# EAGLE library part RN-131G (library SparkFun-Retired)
Roving Netowrks WiFLy GSX Module
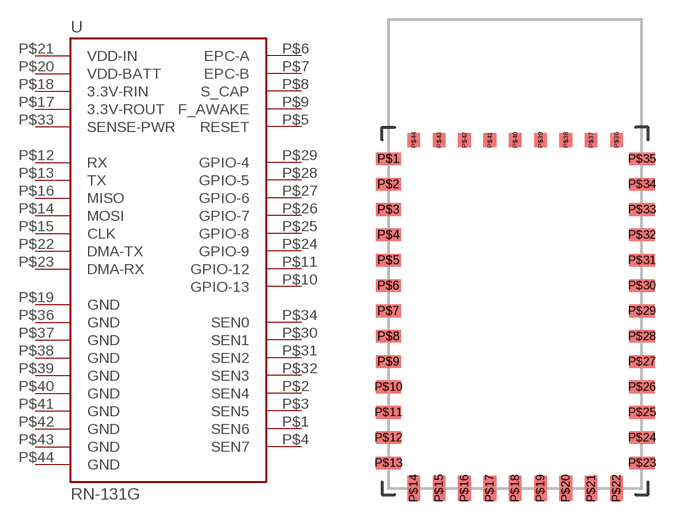
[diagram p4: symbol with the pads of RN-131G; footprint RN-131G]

Designator prefix -

## RN-131G (PROD_ID: IC-12671; SF_ID: WRL-10004)  [RN-131G]
P$1  SEN6
P$2  SEN4
P$3  SEN5
P$4  SEN7
P$5  RESET
P$6  EPC-A
P$7  EPC-B
P$8  S_CAP
P$9  F_AWAKE
P$10  GPIO-13
P$11  GPIO-12
P$12  RX
P$13  TX
P$14  MOSI
P$15  CLK
P$16  MISO
P$17  3.3V-ROUT
P$18  3.3V-RIN
P$19  GND
P$20  VDD-BATT
P$21  VDD-IN
P$22  DMA-TX
P$23  DMA-RX
P$24  GPIO-9
P$25  GPIO-8
P$26  GPIO-7
P$27  GPIO-6
P$28  GPIO-5
P$29  GPIO-4
P$30  SEN1
P$31  SEN2
P$32  SEN3
P$33  SENSE-PWR
P$34  SEN0
P$36  GND
P$37  GND
P$38  GND
P$39  GND
P$40  GND
P$41  GND
P$42  GND
P$43  GND
P$44  GND

## Footprint RN-131G (pad centres in mm)
smd 2 x 1: P$1 -10,11; P$2 -10,9; P$3 -10,7; P$4 -10,5; P$5 -10,3; P$6 -10,1; P$7 -10,-1; P$8 -10,-3; P$9 -10,-5; P$10 -10,-7; P$11 -10,-9; P$12 -10,-11; P$13 -10,-13; P$23 10,-13; P$24 10,-11; P$25 10,-9; P$26 10,-7; P$27 10,-5; P$28 10,-3; P$29 10,-1; P$30 10,1; P$31 10,3; P$32 10,5; P$33 10,7; P$34 10,9; P$35 10,11
smd 1 x 2: P$14 -8,-15; P$15 -6,-15; P$16 -4,-15; P$17 -2,-15; P$18 0,-15; P$19 2,-15; P$20 4,-15; P$21 6,-15; P$22 8,-15
smd 1 x 1.11: P$36 8,12.492; P$37 6,12.492; P$38 4,12.492; P$39 2,12.492; P$40 0,12.492; P$41 -2,12.492; P$42 -4,12.492; P$43 -6,12.492; P$44 -8,12.492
